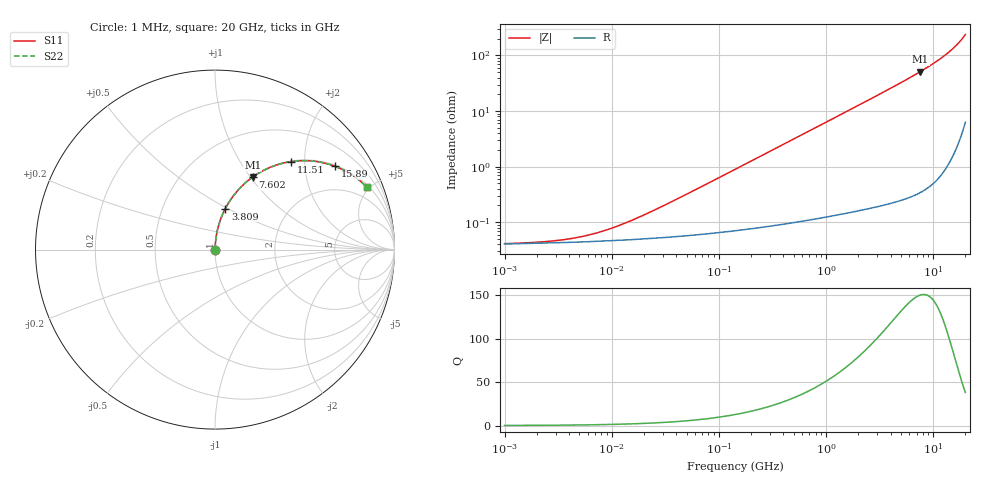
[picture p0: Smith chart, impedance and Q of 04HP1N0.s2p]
# MHz S MA R 50
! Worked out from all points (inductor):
!   216 points, 1 MHz to 20 GHz, reference 50 ohm
!   read as one part in series: L = 1 nH near 25.14 MHz
!   highest Q = 150 at 7.602 GHz (marker M1), where L = 1.07 nH
!   S11 on the Smith chart (normalised r, x): 1 MHz: 1.00, +0.00; 3.809 GHz: 1.00, +0.49; 7.602 GHz: 1.01, +1.03; 11.51 GHz: 1.01, +1.71; 15.89 GHz: 1.04, +2.85; 20 GHz: 1.13, +4.77
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1  0.0004117 8.8  0.9996 -0.0  0.9996 -0.0  0.0004117 8.8
2.63088  0.0004547 21.3  0.9996 -0.0  0.9996 -0.0  0.0004547 21.3
3.80311  0.000494 28.9  0.9996 -0.0  0.9996 -0.0  0.000494 28.9
5.25016  0.0005512 36.7  0.9996 -0.0  0.9996 -0.0  0.0005512 36.7
7.58946  0.0006584 46.4  0.9995 -0.0  0.9995 -0.0  0.0006584 46.4
10.9711  0.0008336 55.7  0.9995 -0.0  0.9995 -0.0  0.0008336 55.7
16.607  0.001152 64.8  0.9995 -0.1  0.9995 -0.1  0.001152 64.8
27.5642  0.001808 73.1  0.9995 -0.1  0.9995 -0.1  0.001808 73.1
144.716  0.009113 85.0  0.9993 -0.5  0.9993 -0.5  0.009113 85.0
759.783  0.04768 85.9  0.9977 -2.7  0.9977 -2.7  0.04768 85.9
1822.98  0.1141 82.7  0.9919 -6.5  0.9919 -6.5  0.1141 82.7
2635.23  0.1644 79.9  0.9846 -9.5  0.9846 -9.5  0.1644 79.9
3809.41  0.2362 75.8  0.9697 -13.7  0.9697 -13.7  0.2362 75.8
3988.98  0.247 75.2  0.9669 -14.3  0.9669 -14.3  0.247 75.2
5766.35  0.3521 69.0  0.9335 -20.6  0.9335 -20.6  0.3521 69.0
7602.03  0.455 62.6  0.8874 -27.1  0.8874 -27.1  0.455 62.6
9570.91  0.5575 55.7  0.8264 -33.9  0.8264 -33.9  0.5575 55.7
11507.3  0.6485 49.1  0.7563 -40.4  0.7563 -40.4  0.6485 49.1
13835.4  0.7436 41.4  0.6615 -48.0  0.6615 -48.0  0.7436 41.4
15885.7  0.8134 34.8  0.5715 -54.4  0.5715 -54.4  0.8134 34.8
18239.8  0.8771 27.6  0.464 -61.3  0.464 -61.3  0.8771 27.6
20000  0.9138 22.5  0.383 -66.0  0.383 -66.0  0.9138 22.5
